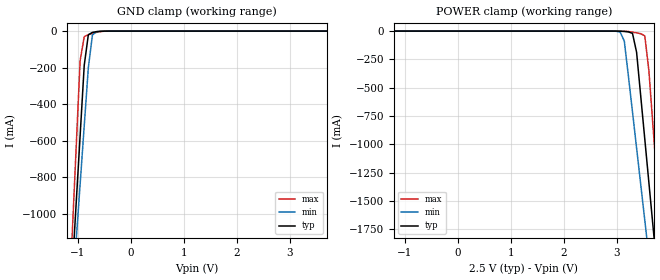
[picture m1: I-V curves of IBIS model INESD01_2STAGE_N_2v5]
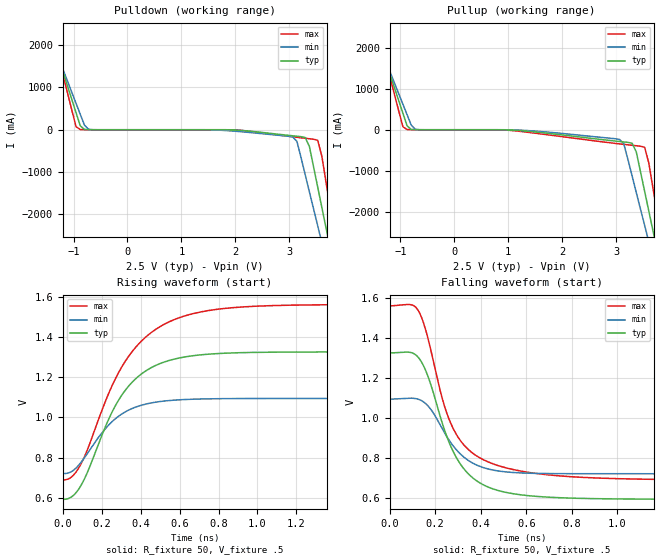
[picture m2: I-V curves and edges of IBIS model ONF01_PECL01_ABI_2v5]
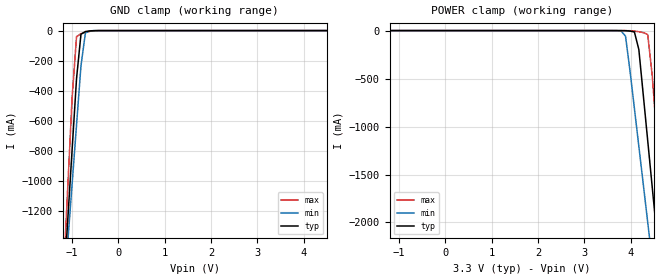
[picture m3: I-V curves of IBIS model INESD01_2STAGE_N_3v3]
|   This file is an IBIS representation of the   |
|   Integrated Devices Technology, Inc.   |
|   ICS843021I-01   |
|   FEMTOCLOCKS CRYSTAL-TO- 3.3V, 2.5V LVPECL CLOCK GENERATOR   |
[IBIS Ver]   4.1
[File name]   843021i_01.ibs
[File Rev]   1.0
[Date]   12 Jan 2009 | Last modified
|   24 Dec 2008 | Generated
[Source]   Originated at Integrated Devices Technology, Inc.
[Disclaimer]
IDT hereby grants the user of this IBIS model a non-exclusive,
nontransferable license to use this IBIS model under the following terms.
Before using this IBIS model, the user should read this license.
If the user does not accept these terms,  the IBIS model should be
returned to IDT within 30 days.
   The user is granted this license only to use the IBIS model and
is not granted rights to sell, load, rent, lease or license the IBIS
model in whole or in part, or in modified form to anyone other than
user. User may modify the IBIS model to suit its specific
applications but rights to derivative works and such modifications
shall belong to IDT.
   This IBIS model is provided on an "AS IS" basis and IDT makes
absolutely no warranty with respect to the information contained
herein. IDT DISCLAIMS AND CUSTOMER WAIVES ALL WARRANTIES, EXPRESS
OR IMPLIED, INCLUDING WARRANTIES OF MERCHANTABILITY OR FITNESS FOR
A PARTICULAR PURPOSE. The entire risk as to quality and performance
is with the Customer. ACCORDINGLY, IN NO EVENT SHALL THE COMPANY BE
LIABLE FOR ANY DAMAGES, WHETHER IN CONTRACT OR TORT,INCLUDING ANY
LOST PROFITS OR OTHER INCIDENTAL, CONSEQUENTIAL, EXEMPLARY, OR
PUNITIVE DAMAGES ARISING OUT OF THE USE OR APPLICATION OF THE IBIS
model provided in this package. Further, IDT reserves the right to
make changes without notice to any product herein to improve
reliability, function, or design. IDT does not convey any license
under patent rights or any other intellectual property rights,
including those of third parties.
   IDT is not obligated to provide maintenance or support
for the licensed IBIS model.
[Copyright]   Copyright 2004 byIntegrated Devices Technology, Inc.
[Component]   ICS843021I-01
[Manufacturer] Integrated Devices Technology, Inc.
[Package]
|TSSOP 8 Lead
|   typ   min   max
R_pkg   52.5m   48.8m   56.2m
L_pkg   1.381nH   1.275nH   1.486nH
C_pkg   0.236pF   0.230pF   0.242pF
[Pin]   signal_name   model_name   R_pin   L_pin   C_pin
1   VCC   POWER   56.2m   1.486n   0.242p
2   VEE   GND   48.8m   1.275n   0.230p
3   XTAL_OUT   NC   48.8m   1.275n   0.230p
4   XTAL_IN   NC   56.2m   1.468n   0.242p
5   OE   INESD01_2STAGE_N   56.2m   1.486n   0.242p
6   VCC   POWER   48.8m   1.275n   0.230p
7   nQ   ONF01_PECL01_ABI   48.8m   1.275n   0.230p
8   Q   ONF01_PECL01_ABI   56.2m   1.468n   0.242p
[Diff Pin]  inv_pin  vdiff tdelay_typ tdelay_min  tdelay_max
8   7   NA   0  0  0
[Model Selector] INESD01_2STAGE_N
INESD01_2STAGE_N_2v5  Buffer selection for 2v5
INESD01_2STAGE_N_3v3  Buffer selection for 3v3
[Model Selector] ONF01_PECL01_ABI
ONF01_PECL01_ABI_2v5  Buffer selection for 2v5
ONF01_PECL01_ABI_3v3  Buffer selection for 3v3
| Models and submodels in the file (4): INESD01_2STAGE_N_2v5 (Input), ONF01_PECL01_ABI_2v5 (Output_ECL), INESD01_2STAGE_N_3v3 (Input), ONF01_PECL01_ABI_3v3 (Output_ECL)
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[Model] INESD01_2STAGE_N_2v5
Model_type   Input
Polarity   Non-Inverting
Vinl = 0.7V
Vinh = 1.7V
|   typ   min   max
C_comp   2pF   1.5pF   2.5pF
|   typ   min   max
[Voltage range]  2.5V   2.375V   2.625V
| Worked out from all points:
|   GND clamp passes 1 mA (typ) near -0.56 V on its own axis
[GND_clamp]
|Voltage   I(typ)   I(min)   I(max)
-2.5V     -8.269A    -7.245A    -9.986A
-1.108V   -1.338A    -1.475A    -1.143A
-1.031V   -954.2mA   -1.155A    -652.3mA
-953.6mV  -570.3mA   -836.3mA   -161.2mA
-876.3mV  -186.9mA   -517.8mA   -30.2mA
-799mV    -20.08mA   -199.8mA   -19.87mA
-721.6mV  -7.049mA   -21.01mA   -12.75mA
-644.3mV  -3.148mA   -2.874mA   -6.745mA
-489.7mV  -290.5uA   -172.1uA   -617.5uA
5V        48.47uA    63.64uA    35.68uA
[POWER_clamp]
|Voltage   I(typ)   I(min)   I(max)
-2.5V     48.47uA    60.61uA    37.56uA
3.067V    -1.084mA   -9.257mA   -231.1uA
3.144V    -3.149mA   -87.7mA    -1.112mA
3.299V    -20.08mA   -714.1mA   -8.879mA
3.376V    -186.9mA   -1.033A    -15.37mA
3.454V    -570.3mA   -1.352A    -22.95mA
3.531V    -954.2mA   -1.672A    -42.3mA
3.608V    -1.338A    -1.991A    -349.4mA
3.686V    -1.723A    -2.311A    -840.5mA
3.763V    -2.108A    -2.632A    -1.332A
3.84V     -2.492A    -2.952A    -1.823A
5V        -8.269A    -7.765A    -9.192A
[Model] ONF01_PECL01_ABI_2v5
Model_type  Output_ECL
Polarity   Non-Inverting
Vmeas = .975
Rref = 50
Cref = 0
Vref = .5
|Variable  typ   min   max
C_comp   2p   1.5p   2.5p
[Voltage Range]   2.5   2.375   2.625
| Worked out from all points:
|   rising waveform, R_fixture 50, V_fixture .5: 20-80 % time 228ps typ, 199ps min, 276ps max; typ from 0.592 V to 1.33 V
|   falling waveform, R_fixture 50, V_fixture .5: 20-80 % time 153ps typ, 140ps min, 156ps max; typ from 1.33 V to 0.592 V
| Open source, no load
|  Voltage   I(typ)   I(min)   I(max)
[Pullup]
-2.5V     6.581A     5.758A     7.966A
-1.572V   2.868A     2.671A     3.219A
-1.418V   2.25A      2.158A     2.429A
-953.6mV  402.1mA    621.9mA    72.14mA
-876.3mV  95.6mA     366.6mA    5.897mA
-721.6mV  951.4uA    9.59mA     751.4uA
3.067V    -287.8mA   -237.7mA   -346mA
3.299V    -330.4mA   -1.134A    -380.1mA
3.531V    -1.506A    -2.34A     -427.9mA
3.686V    -2.47A     -3.144A    -1.427A
3.84V     -3.434A    -3.947A    -2.655A
5V        -10.66A    -9.976A    -11.86A
[Pulldown]
-2.5V     6.581A     5.758A     7.966A
-1.495V   2.559A     2.415A     2.824A
-1.418V   2.25A      2.158A     2.429A
-953.6mV  402.1mA    621.9mA    72.14mA
-876.3mV  95.6mA     366.6mA    5.897mA
-721.6mV  951.4uA    9.59mA     751.4uA
3.067V    -142.9mA   -171.4mA   -166.7mA
3.299V    -185mA     -1.067A    -201.5mA
3.531V    -1.361A    -2.272A    -250mA
3.686V    -2.324A    -3.076A    -1.249A
3.84V     -3.288A    -3.879A    -2.478A
5V        -10.51A    -9.904A    -11.69A
[Ramp]
|   typ   min   max
dV/dt_r   0.586/0.368n   0.299/0.313n   0.698/0.446n
dV/dt_f   0.590/0.258n   0.302/0.226n   0.703/0.290n
R_load =   50.0000
[Rising Waveform]
R_fixture = 50
V_fixture = .5   | VCC_typ - 2V
V_fixture_max = 0.625   | VCC_max - 2V
V_fixture_min = 0.375   | VCC_min - 2V
C_fixture = 0.0p
| Time   typ   min   max
0s        592.5mV    720.8mV    689.3mV
46.2ps    605.5mV    731.1mV    704.8mV
92.4ps    659.4mV    774.5mV    766.4mV
241.5ps   1.003V     967.6mV    1.133V
323.4ps   1.138V     1.029V     1.283V
426.3ps   1.231V     1.066V     1.4V
552.3ps   1.285V     1.084V     1.478V
711.9ps   1.312V     1.092V     1.525V
940.8ps   1.323V     1.094V     1.551V
1.999ns   1.326V     1.094V     1.562V
[Falling Waveform]
R_fixture = 50
V_fixture = .5   | VCC_typ - 2V
V_fixture_max = 0.625   | VCC_max - 2V
V_fixture_min = 0.375   | VCC_min - 2V
C_fixture = 0.0p
| Time   typ   min   max
0s        1.326V     1.094V     1.562V
92.4ps    1.328V     1.099V     1.568V
123.9ps   1.306V     1.095V     1.541V
168ps     1.209V     1.061V     1.4V
231ps     973.8mV    945.4mV    1.097V
277.2ps   835.9mV    862.7mV    951mV
348.6ps   716.5mV    784.8mV    838.7mV
447.3ps   647.2mV    740.6mV    773mV
865.2ps   596.5mV    720.8mV    701.4mV
1.999ns   592.4mV    720.7mV    689.3mV
[Model] INESD01_2STAGE_N_3v3
Model_type   Input
Polarity   Non-Inverting
Vinl = 0.8V
Vinh = 2.0V
|   typ   min   max
C_comp   2pF   1.5pF   2.5pF
|   typ   min   max
[Voltage range]  3.3V   3.15V   3.45V
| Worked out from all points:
|   GND clamp passes 1 mA (typ) near -0.55 V on its own axis
[GND_clamp]
|Voltage   I(typ)   I(min)   I(max)
-3.3V     -12.25A    -10.57A    -15.07A
-1.191V   -1.749A    -1.815A    -1.667A
-1.095V   -1.272A    -1.419A    -1.058A
-999mV    -795.5mA   -1.023A    -449.3mA
-903.1mV  -319.8mA   -628.1mA   -40.47mA
-807.2mV  -23.98mA   -233.7mA   -20.7mA
-711.3mV  -6.373mA   -15.69mA   -11.88mA
-615.5mV  -2.208mA   -1.554mA   -4.927mA
-519.6mV  -502.9uA   -282.7uA   -1.127mA
6V        52.35uA    69.46uA    38.08uA
[POWER_clamp]
|Voltage   I(typ)   I(min)   I(max)
-3.3V     63.98uA    80.01uA    49.58uA
3.795V    -332uA     -4.132mA   -63.8uA
3.891V    -1.568mA   -57.73mA   -179.8uA
3.987V    -4.988mA   -416.2mA   -1.17mA
4.082V    -14.84mA   -811mA     -5.045mA
4.178V    -197.1mA   -1.206A    -12.05mA
4.37V     -1.149A    -1.999A    -41.75mA
4.466V    -1.626A    -2.396A    -462.1mA
4.562V    -2.102A    -2.793A    -1.071A
4.658V    -2.58A     -3.19A     -1.68A
4.754V    -3.057A    -3.588A    -2.29A
6V        -9.266A    -8.761A    -10.21A
